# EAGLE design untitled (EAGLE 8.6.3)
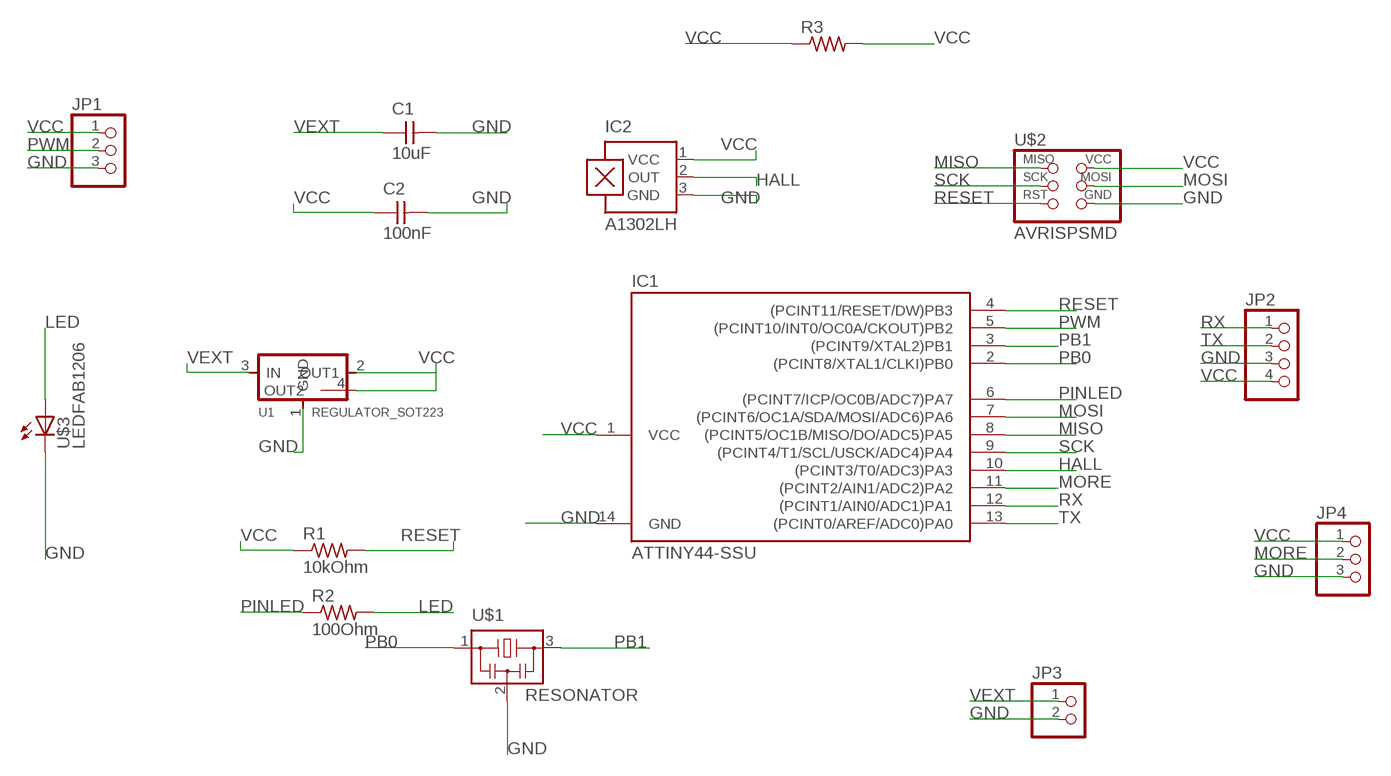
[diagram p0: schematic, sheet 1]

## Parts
C1  10uF  CAP-UNPOLARIZEDFAB  [C1206FAB]
C2  100nF  CAP-UNPOLARIZEDFAB  [C1206FAB]
IC1  ATTINY44-SSU  [SOIC14]
IC2  A1302LH  [SOT23-W]
JP1  PINHD-1X3  [1X03]
JP2  PINHD-1X4  [1X04]
JP3  PINHD-1X2  [1X02]
JP4  PINHD-1X3  [1X03]
R1  10kOhm  RES-US1206FAB  [R1206FAB]
R2  100Ohm  RES-US1206FAB  [R1206FAB]
R3  RES-US1206FAB  [R1206FAB]
U1  REGULATOR_SOT223  [SOT223]
U$1  RESONATOR  [EFOBM]
U$2  AVRISPSMD  [2X03SMD]
U$3  LEDFAB1206  [LED1206FAB]

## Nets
GND: C1.2 C2.2 IC1.14(GND) IC2.3(GND) JP1.3 JP2.3 JP3.2 JP4.3 U1.1(GND) U$1.2 U$2.6(GND) U$3.2(C)
HALL: IC1.10((PCINT3/T0/ADC3)PA3) IC2.2(OUT)
LED: R2.2 U$3.1(A)
MISO: IC1.8((PCINT5/OC1B/MISO/DO/ADC5)PA5) U$2.1(MISO)
MORE: IC1.11((PCINT2/AIN1/ADC2)PA2) JP4.2
MOSI: IC1.7((PCINT6/OC1A/SDA/MOSI/ADC6)PA6) U$2.4(MOSI)
PB0: IC1.2((PCINT8/XTAL1/CLKI)PB0) U$1.1
PB1: IC1.3((PCINT9/XTAL2)PB1) U$1.3
PINLED: IC1.6((PCINT7/ICP/OC0B/ADC7)PA7) R2.1
PWM: IC1.5((PCINT10/INT0/OC0A/CKOUT)PB2) JP1.2
RESET: IC1.4((PCINT11/RESET/DW)PB3) R1.2 U$2.5(RST)
RX: IC1.12((PCINT1/AIN0/ADC1)PA1) JP2.1
SCK: IC1.9((PCINT4/T1/SCL/USCK/ADC4)PA4) U$2.3(SCK)
TX: IC1.13((PCINT0/AREF/ADC0)PA0) JP2.2
VCC: C2.1 IC1.1(VCC) IC2.1(VCC) JP1.1 JP2.4 JP4.1 R1.1 R3.1 R3.2 U1.2(OUT1) U1.4(OUT2) U$2.2(VCC)
VEXT: C1.1 JP3.1 U1.3(IN)

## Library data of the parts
C1 C2 = 001_fab:CAP-UNPOLARIZED
IC1 = 001_fab:ATTINY44
IC2 = allegro:A13*?: Linear Hall Effect Sensor ICs Continuous-Time Ratiometric High-Temperature Operation Programmable Linear with Analog Output A1302 -Replacement- UGN3503 Source: http://www.allegromicro.com/en/Products/Part_Numbers/1301/1301.pdf http://www.allegromicro.com/en/Products/Part_Numbers/1321/1321.pdf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; MF: ALLEGRO MICROSYSTEMS, INC.; MPN: A1302ELHLT-T; OC_FARNELL: 1457209; OC_NEWARK: 31K6638
JP1 JP4 = pinhead:PINHD-1X3: PIN HEADER
JP2 = pinhead:PINHD-1X4: PIN HEADER
JP3 = pinhead:PINHD-1X2: PIN HEADER
R1-R3 = 001_fab:RES-US: Resistor (US Symbol)
U1 = 001_fab:REGULATOR_SOT223
U$1 = 001_fab:RESONATOR
U$2 = 001_fab:AVRISP
U$3 = 001_fab:LED: LED

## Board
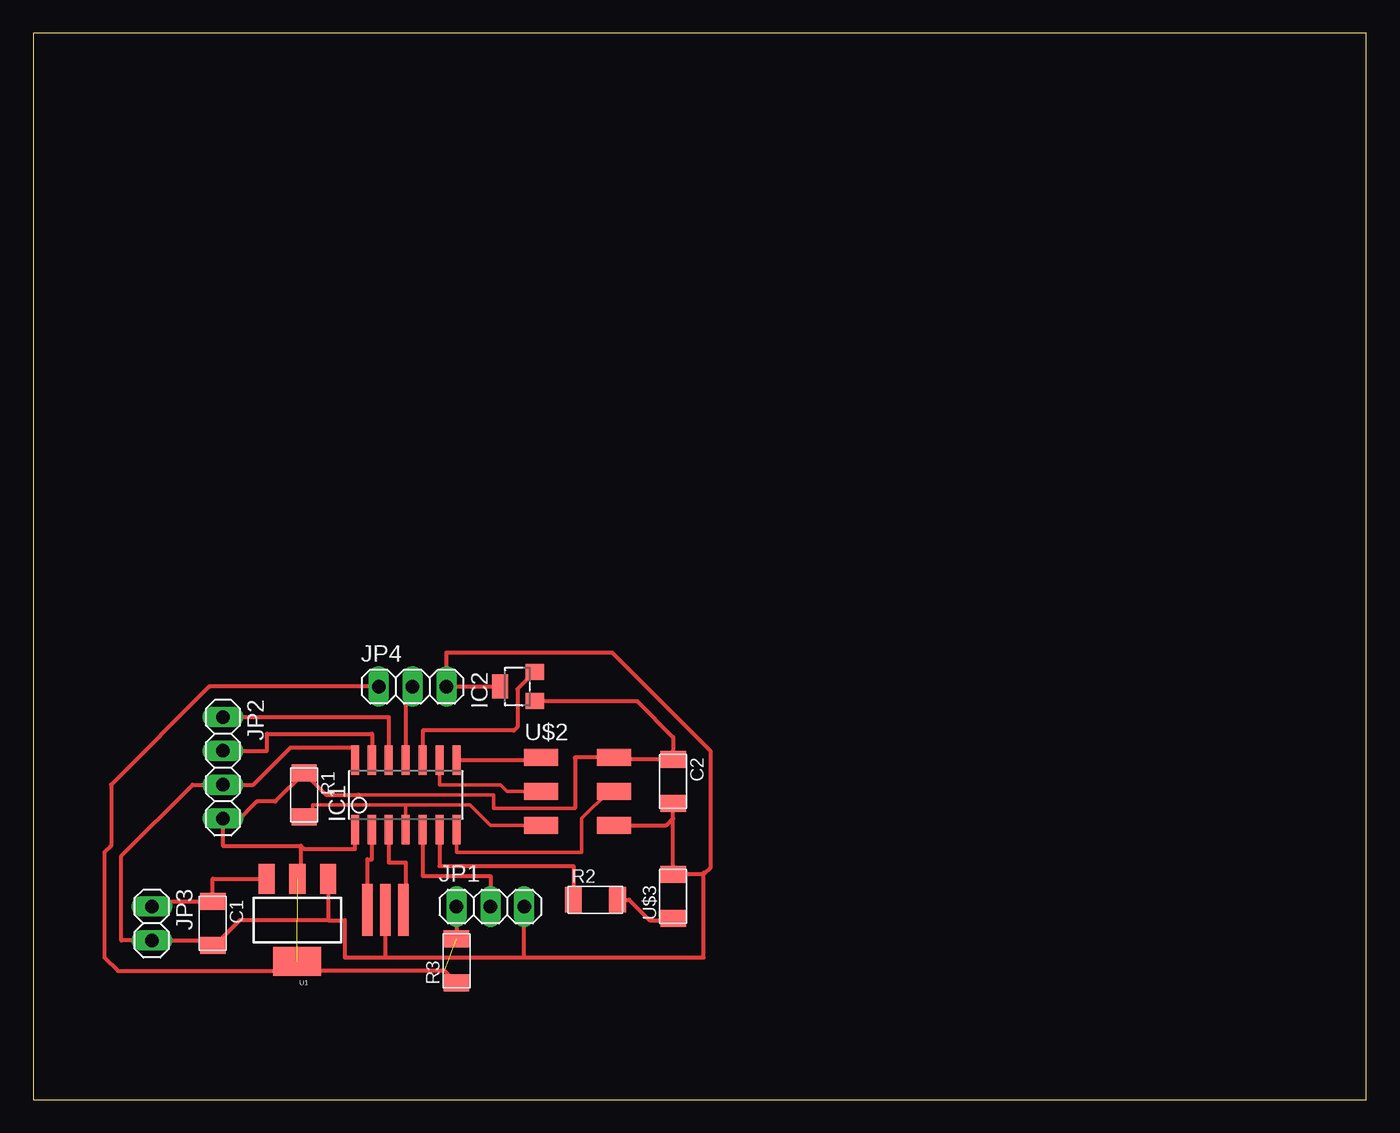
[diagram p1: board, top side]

Size 100 x 80 mm. Coordinates in mm from the lower left corner, seen from the top.
Outline: 0,0 100,0 100,80 0,80 0,0
Copper layers (1*16): Top 0.035mm / dielectric 1.5mm / Bottom 0.035mm
Design rules "default": minimum track width 6mil, minimum drill 0.35mm, track to track 6mil, track to pad 6mil, pad to pad 6mil, via to via 6mil, smd to smd 6mil, copper to edge 40mil, drill to drill 6mil, minimum pad ring 10mil, minimum via ring 8mil, stop-mask expansion 4mil, vias tented up to drill 0mil, thermal gap 10mil

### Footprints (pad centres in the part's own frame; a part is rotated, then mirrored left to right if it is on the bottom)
C1206FAB = smd 1.27 x 1.905: 1 -1.651,0; 2 1.651,0
SOIC14 = smd 0.61 x 2.21: 1 -3.81,-2.603; 2 -2.54,-2.603; 3 -1.27,-2.603; 4 0,-2.603; 5 1.27,-2.603; 6 2.54,-2.603; 7 3.81,-2.603; 8 3.81,2.603; 9 2.54,2.603; 10 1.27,2.603; 11 0,2.603; 12 -1.27,2.603; 13 -2.54,2.603; 14 -3.81,2.603
SOT23-W = smd 1.2 x 1.4: 1 -1.1,-1.3; 2 1.1,-1.3 | smd 1.8 x 1.2: 3 0,1.3
1X03 = drill 1.016 long: 1 -2.54,0; 2 0,0; 3 2.54,0
1X04 = drill 1.016 long: 1 -3.81,0; 2 -1.27,0; 3 1.27,0; 4 3.81,0
1X02 = drill 1.016 long: 1 -1.27,0; 2 1.27,0
R1206FAB = smd 1.27 x 1.905: 1 -1.651,0; 2 1.651,0
SOT223 = smd 1.219 x 2.235: 1 -2.311,-3.099; 2 0,-3.099; 3 2.311,-3.099 | smd 3.6 x 2.2: 4 0,3.099
EFOBM = smd 0.8 x 3.9: 1 -1.35,0; 2 0,0; 3 1.35,0
2X03SMD = smd 2.54 x 1.27: 1 -2.54,2.54; 2 2.92,2.54; 3 -2.54,0; 4 2.92,0; 5 -2.54,-2.54; 6 2.92,-2.54
LED1206FAB = smd 1.27 x 1.905: 1 -1.651,0; 2 1.651,0

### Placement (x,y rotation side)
C1  13.46,13.21 270 top
C2  48.01,23.88 270 top
IC1  27.94,22.86 0 top
IC2  36.32,30.99 90 top
JP1  34.29,14.48 0 top
JP2  14.22,24.89 270 top
JP3  8.89,13.21 270 top
JP4  28.45,30.99 0 top
R1  20.32,22.86 270 top
R2  42.16,14.99 0 top
R3  31.75,10.41 90 top
U1  19.81,13.46 180 top
U$1  26.42,14.22 0 top
U$2  40.64,23.11 0 top
U$3  48.01,15.24 90 top

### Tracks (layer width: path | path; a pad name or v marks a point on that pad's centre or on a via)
GND
  Top 0.305: IC2.3 JP4.3 30.99,33.53 33.53,33.53 33.78,33.53 43.43,33.53 50.8,26.16 50.8,17.4 50.29,16.89 | U$2.6 47.5,20.57 48.01,21.08 | 48.01,21.08 C2.2 | U1.1 22.12,13.46 | 22.12,13.46 15.49,13.46 13.59,11.56 C1.2 13.46,11.94 JP3.2 6.6,11.94 6.6,18.29 11.94,23.62 JP2.3 16.51,23.62 19.3,26.42 24.13,26.42 IC1.14 | 22.12,13.46 23.37,13.46 23.37,10.67 26.42,10.67 | 26.42,10.67 U$1.2 | 26.42,10.67 36.83,10.67 | 36.83,10.67 JP1.3 | 36.83,10.67 50.29,10.67 50.29,16.89 | 50.29,17.02 50.29,16.89 | 50.29,16.89 U$3.2 48.01,21.08
HALL
  Top 0.305: IC2.2 36.32,30.79 36.32,27.94 36.07,27.69 29.21,27.69 IC1.10
LED
  Top 0.305: R2.2 44.7,14.99 46.23,13.46 47.88,13.46 U$3.1
MISO
  Top 0.305: IC1.8 37.91,25.46 U$2.1
MORE
  Top 0.305: JP4.2 27.94,30.48 IC1.11
MOSI
  Top 0.254: IC1.7 31.75,18.54 41.15,18.54 41.15,21.08 43.18,23.11 U$2.4
PB0
  Top 0.305: U$1.1 25.07,18.03 25.4,18.03 IC1.2
PB1
  Top 0.305: IC1.3 26.67,17.78 27.94,17.78 27.94,14.22 U$1.3
PINLED
  Top 0.305: IC1.6 30.48,17.53 40.51,17.53 R2.1
PWM
  Top 0.305: IC1.5 29.21,16.76 34.29,16.76 JP1.2
RESET
  Top 0.254: R1.2 20.95,21.84 20.95,22.1 27.94,22.1 | U$2.5 34.29,20.57 32.77,22.1 27.94,22.1 | 27.94,22.1 IC1.4
RX
  Top 0.305: JP2.1 26.67,28.7 IC1.12
SCK
  Top 0.254: U$2.3 35.56,23.11 35.05,23.62 30.48,23.62 IC1.9
TX
  Top 0.305: JP2.2 17.53,26.16 17.53,27.43 25.4,27.43 IC1.13
VCC  (2 unrouted)
  Top 0.254: 40.64,21.84 34.54,21.84 34.54,22.86 24.38,22.86 24.13,22.86
  Top 0.305: 40.64,21.84 40.64,25.65 U$2.2 43.56,25.53 C2.1 48.01,27.18 45.3,29.89 IC2.1 | 24.38,22.86 21.97,22.86 R1.1 18.16,22.35 16.76,22.35 15.24,20.83 14.48,20.83 JP2.4 14.22,19.05 20.07,19.05 | 20.07,19.05 20.07,16.56 U1.2 | JP1.1 R3.2 | R3.1 30.86,9.65 19.05,9.65 19.76,10.36 U1.4 19.1,9.65 6.35,9.65 5.33,10.67 5.33,18.54 5.84,19.05 5.84,23.62 13.21,30.99 JP4.1 | 20.07,19.05 20.32,18.8 24.13,18.8 IC1.1
VEXT
  Top 0.305: JP3.1 8.89,14.86 C1.1 13.46,16.56 U1.3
